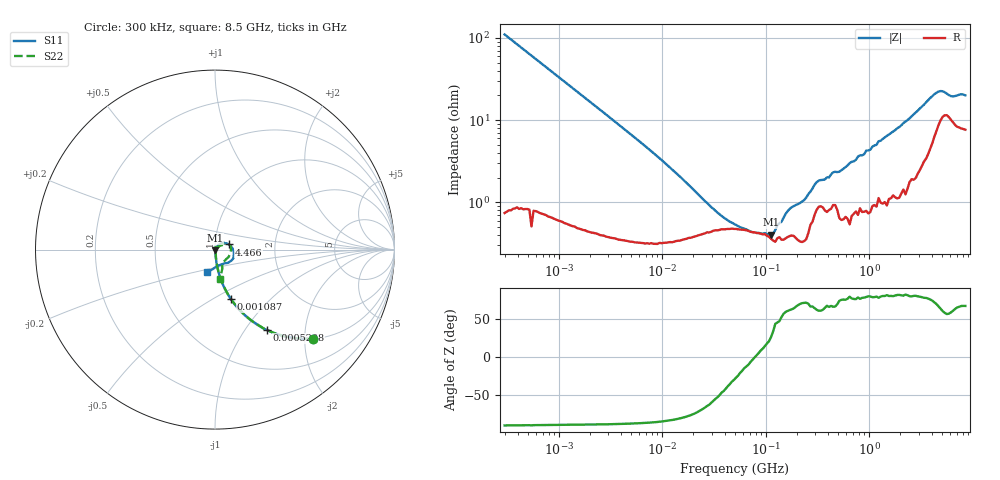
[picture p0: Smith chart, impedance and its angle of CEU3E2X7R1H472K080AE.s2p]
! S-parameter Generated by TDK Corporation
! Copyright(C) 2015 TDK Corporation.
! All Rights Reserved.
! TDK P/N: CEU3E2X7R1H472K080AE (Multilayer Ceramic Chip Capacitors)
! Property: C=4.7nF
! Size(LxWxT): 1.6x0.8x0.8mm, 0.063x0.031x0.031inches
! Model Type: s2p (Touchstone File Format Version 1.0)
! Frequency: DC=Yes Start=0.3MHz Stop=8500MHz 225points Log-sweep
! Note:
! Model Generated on Jun. 23, 2015
! Hash(MD5):
! Port Assignments:
!  1 ---| |--- 2
! Applicable Conditions:
!  Temperature = 25 degC
!  DC Bias Voltage = 0 V
!  Small Signal Operation
! Terms and conditions regarding TDK Simulation Models
! (1)This simulation model is being provided solely for informational purposes. Please refer to the specifications of the products in terms of detailed characteristics of such products.
! (2)In no event shall TDK Corporation of any of its subsidiaries be liable for any loss or damage arising, directly or indirectly,
!  From any information contained in this simulation model, including, but not limited to loss or damages arising from any inaccuracies, omissions or errors in connection with such information.
! (3)Any and all copyrights on this simulation model are owned by TDK Corporation.
!  Duplication or redistribution of this simulation model without prior written permission from TDK Corporation is prohibited.
! (4)This simulation model is subject to any modification or change without any prior notice.
! (5)Neither TDK Corporation nor any of its subsidiaries shall make any warranty, express or implied,
!  Including but not limited to the correctness, implied warranties of merchantability and fitness for a particular purpose with respect to this simulation models.
! (6)The use of this simulation model shall be deemed to have consented to the terms and conditions hereof.
# MHz S MA R 50
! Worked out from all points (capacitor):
!   224 points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, 300 kHz to 8.5 GHz, reference 50 ohm
!   read as one part in series: C = 4.81 nF near 314.1 kHz
!   lowest |Z| = 403 mohm at 112.9 MHz (marker M1)
!   series resonance near 78.29 MHz, so ESL is about 860 pH
!   S11 on the Smith chart (normalised r, x): 300 kHz: 1.01, -2.20; 520.8 kHz: 1.01, -1.27; 1.087 MHz: 1.01, -0.61; 4.466 GHz: 1.16, +0.07; 8.5 GHz: 0.89, -0.23
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0.3  0.7383 -42.1  0.6703 47.4  0.672 47.6  0.7374 -42.2
0.5208429  0.5336 -57.1  0.8384 32.2  0.8389 32.3  0.5332 -57.1
1.086811  0.2917 -72.0  0.9509 17.0  0.9511 17.0  0.2916 -72.0
1.72111  0.1899 -77.7  0.9772 10.9  0.9774 11.0  0.1899 -77.7
9.430415  0.03437 -83.6  0.9958 1.9  0.9963 1.9  0.03462 -82.4
51.67171  0.002426 -84.5  0.9934 -0.0  0.9937 -0.0  0.0099 -54.1
112.8926  0.003052 -105.1  0.9921 -0.4  0.9927 -0.4  0.004517 -92.4
148.7505  0.001649 -72.1  0.9929 -0.7  0.9933 -0.6  0.0006627 126.8
170.7477  0.0004849 -163.2  0.9923 -0.8  0.9928 -0.8  0.001322 35.1
195.9978  0.001986 179.6  0.9915 -1.0  0.992 -0.9  0.0005466 72.8
283.1228  0.00529 -34.5  0.9898 -1.4  0.9904 -1.3  0.009697 96.2
469.456  0.01136 49.7  0.9891 -2.2  0.9898 -2.2  0.008645 1.5
514.6664  0.009935 76.1  0.9886 -2.4  0.989 -2.3  0.001783 -52.5
564.2308  0.007063 67.2  0.9895 -2.5  0.9901 -2.5  0.005265 66.7
647.669  0.008517 81.2  0.9888 -3.0  0.9893 -3.0  0.003957 106.0
710.042  0.003207 62.4  0.9879 -3.2  0.9884 -3.2  0.00939 63.5
815.0429  0.01052 73.3  0.9863 -3.7  0.9867 -3.7  0.006956 48.4
1025.67  0.003625 45.3  0.9868 -4.6  0.9878 -4.6  0.00789 66.7
1232.735  0.01286 41.7  0.9853 -5.6  0.9857 -5.6  0.01448 55.2
1551.304  0.01175 53.7  0.9834 -7.0  0.984 -6.9  0.01202 55.0
4465.833  0.08218 20.5  0.9202 -20.0  0.921 -20.0  0.08204 20.9
8500  0.1322 -108.8  0.9019 -30.8  0.9025 -30.9  0.1667 -80.5
